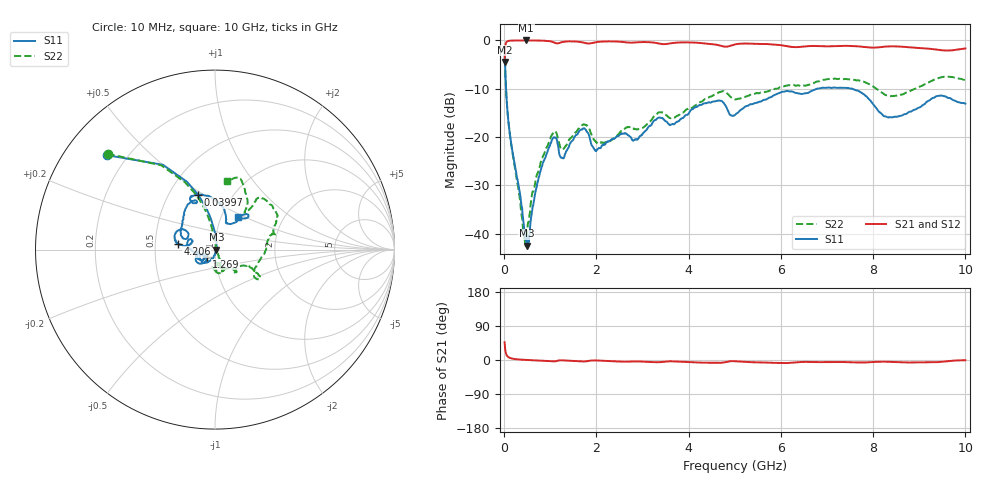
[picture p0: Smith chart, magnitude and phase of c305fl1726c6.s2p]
!Agilent Technologies,N5234A,MY52241123,A.10.00.00
!Agilent N5234A: A.10.00.00
!Date: Tuesday, October 22, 2019 08:06:12
!Correction: S11(Full 2 Port(1,2))
!S21(Full 2 Port(1,2))
!S12(Full 2 Port(1,2))
!S22(Full 2 Port(1,2))
!S2P File: Measurements: S11, S21, S12, S22:
# Hz S  dB  R 50
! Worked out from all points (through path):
!   1001 points, 10 MHz to 10 GHz, reference 50 ohm
!   highest |S21| = -0.02 dB at 479.5 MHz (marker M1); lowest = -4.5 dB at 10 MHz (marker M2)
!   lowest |S11| = -42.5 dB at 489.5 MHz (marker M3), VSWR 1.02, Z = 50.8 + j0.0198 ohm
!   |S11| at or under -10 dB: 40.51 MHz to 6.785 GHz (6.745 GHz wide, 198 % of centre); 7.545 GHz to end of sweep
!   |S22| runs from -42.6 to -1.9 dB; largest |S21 - S12| = 0.0023
!   S11 on the Smith chart (normalised r, x): 10 MHz: 0.13, +0.37; 39.97 MHz: 0.70, +0.47; 1.269 GHz: 0.91, -0.07; 4.206 GHz: 0.65, +0.04; 10 GHz: 1.21, +0.45
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1e7  -1.94 138.9  -4.49 47.1  -4.47 47.0  -1.92 138.3
3.997e7  -9.90 107.2  -0.53 17.1  -0.54 17.2  -9.87 108.8
7.993e7  -15.55 97.2  -0.16 8.8  -0.16 8.8  -15.56 100.7
1.4986e8  -21.15 89.4  -0.06 4.5  -0.07 4.5  -21.29 96.0
4.1959e8  -37.67 50.5  -0.02 0.5  -0.03 0.6  -39.38 52.1
4.7953e8  -41.66 11.9  -0.02 0.2  -0.03 0.2  -41.51 -5.0
4.8952e8  -42.45 1.5  -0.03 0.1  -0.03 0.1  -40.76 -16.0
6.5935e8  -32.20 -92.1  -0.04 -0.9  -0.04 -0.9  -30.25 -60.5
1.01899e9  -21.07 -124.6  -0.24 -3.5  -0.25 -3.6  -19.84 -72.3
1.26874e9  -24.33 -140.6  -0.34 -0.8  -0.34 -0.8  -22.61 -82.9
1.67833e9  -18.46 -140.6  -0.38 -3.7  -0.37 -3.7  -17.69 -70.1
2.008e9  -22.74 -147.0  -0.36 -1.3  -0.37 -1.3  -21.20 -83.6
3.34666e9  -15.98 168.2  -0.64 -5.9  -0.65 -5.9  -14.93 -46.3
3.64636e9  -17.34 163.3  -0.57 -3.6  -0.57 -3.5  -15.90 -40.8
4.2058e9  -13.51 171.4  -0.51 -6.6  -0.52 -6.6  -13.12 -26.8
4.68532e9  -12.48 156.5  -1.08 -7.5  -1.09 -7.5  -10.66 -31.3
5.005e9  -15.42 159.2  -0.83 -3.2  -0.84 -3.3  -12.21 -26.2
6.67333e9  -10.42 115.9  -1.16 -5.3  -1.17 -5.3  -8.92 21.8
7.64236e9  -10.33 98.9  -1.22 -6.5  -1.22 -6.5  -8.28 48.0
8.34166e9  -15.90 66.9  -1.24 -4.9  -1.24 -4.9  -11.47 51.0
9.42058e9  -11.47 47.4  -1.97 -5.5  -1.98 -5.5  -7.78 68.5
1e10  -13.09 53.9  -1.68 -0.7  -1.68 -0.8  -8.24 79.9
